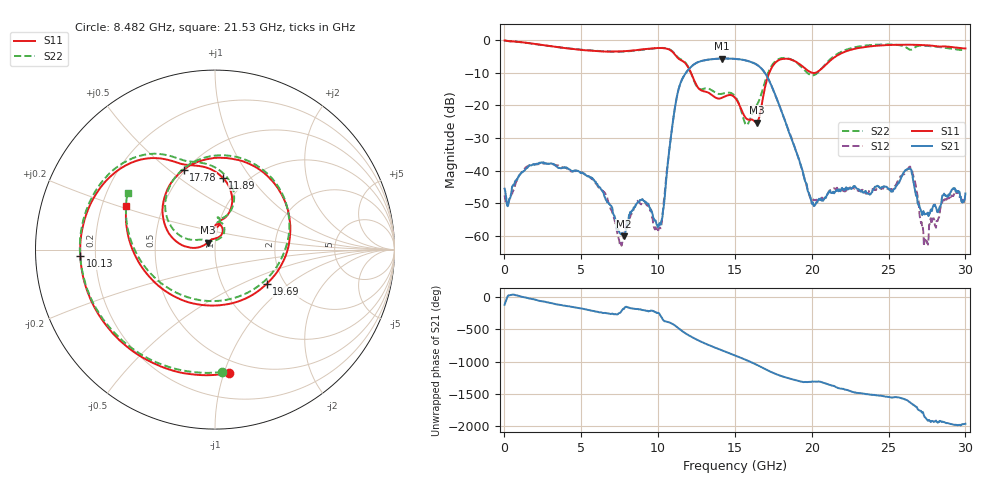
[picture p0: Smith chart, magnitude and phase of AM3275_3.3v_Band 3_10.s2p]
!Keysight Technologies,N5245B,MY58422270,A.16.20.02
!Date: Thursday, March 27, 2025 02:01:57
!Correction: S11(C  2-Port  )
!S21(C  2-Port  )
!S12(C  2-Port  )
!S22(C  2-Port  )
!S2P File: Measurements: S11, S21, S12, S22:
# Hz S  dB  R 50
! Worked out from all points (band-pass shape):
!   801 points, 10 MHz to 30 GHz, reference 50 ohm
!   highest |S21| = -5.71 dB at 14.14 GHz (marker M1); lowest = -60.1 dB at 7.77 GHz (marker M2)
!   |S21| within 3 dB of the highest: 12.05 GHz to 16.71 GHz (4.667 GHz wide, 32.5 % of centre)
!   lowest |S11| = -25.3 dB at 16.43 GHz (marker M3), VSWR 1.11, Z = 46.2 + j3.59 ohm
!   |S11| at or under -10 dB: 12.13 GHz to 17.24 GHz (5.114 GHz wide, 34.8 % of centre); 19.99 GHz to 20.28 GHz (292.2 MHz wide, 1.45 % of centre)
!   |S22| runs from -26.1 to -0.2 dB; largest |S21 - S12| = 0.0095
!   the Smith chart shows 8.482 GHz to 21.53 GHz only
!   S11 on the Smith chart (normalised r, x): 8.482 GHz: 0.39, -1.04; 10.13 GHz: 0.14, -0.02; 11.89 GHz: 0.78, +0.74; 17.78 GHz: 0.49, +0.56; 19.69 GHz: 1.62, -0.70; 21.53 GHz: 0.30, +0.21
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1e7  -0.18 -3.6  -45.55 -118.7  -47.59 60.5  -0.18 -4.6
1.284575e9  -0.80 -81.4  -40.03 -3.2  -39.59 -2.4  -0.83 -82.0
2.671612e9  -1.72 -158.3  -37.76 -74.5  -37.80 -77.7  -1.74 -159.6
5.033325e9  -3.09 90.5  -40.79 179.9  -40.51 -177.2  -3.01 88.6
7.769912e9  -3.49 -44.6  -60.08 174.3  -60.14 -173.1  -3.56 -47.2
8.482175e9  -3.19 -83.7  -51.14 177.0  -51.22 -178.6  -3.31 -86.7
1.001916e10  -2.49 -170.7  -56.69 115.3  -58.23 86.2  -2.49 -173.7
1.013162e10  -2.49 -177.4  -56.39 78.9  -57.44 33.1  -2.46 179.8
1.114379e10  -4.80 119.0  -19.36 -88.6  -19.33 -88.8  -4.62 116.6
1.189354e10  -7.89 83.9  -9.56 142.3  -9.55 142.3  -7.71 81.1
1.305565e10  -15.81 81.0  -6.22 1.6  -6.21 1.7  -14.84 85.5
1.414279e10  -17.74 89.4  -5.71 -103.2  -5.72 -103.3  -16.52 84.7
1.5005e10  -17.73 72.3  -5.81 176.9  -5.80 176.9  -17.25 68.1
1.642952e10  -25.30 134.5  -7.61 31.7  -7.61 31.6  -19.94 146.5
1.777908e10  -6.42 111.6  -18.66 -121.0  -18.70 -121.1  -6.04 105.7
1.969094e10  -9.23 -33.6  -44.59 124.4  -45.19 121.6  -10.01 -40.0
2.002832e10  -10.06 -71.6  -50.28 133.1  -49.09 137.7  -10.86 -82.0
2.152782e10  -5.17 153.6  -46.53 53.8  -45.65 53.8  -4.71 147.0
2.501416e10  -1.58 38.7  -45.64 -104.0  -45.73 -102.8  -1.39 35.0
2.643869e10  -1.49 3.5  -39.54 164.0  -39.17 164.3  -3.04 2.8
2.745085e10  -1.65 -23.4  -53.20 -81.8  -60.87 -80.8  -1.82 -23.6
3e10  -2.61 -111.9  -46.99 -158.0  -49.19 -164.9  -3.09 -114.8
